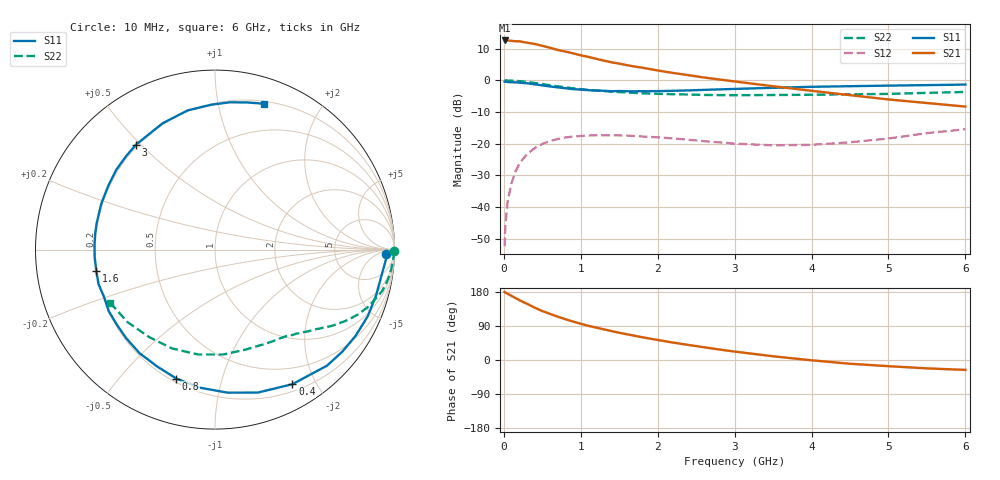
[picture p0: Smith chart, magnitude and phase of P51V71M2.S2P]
! SIEMENS Small Signal Semiconductors
! BFP183
! Si NPN RF Bipolar Junction Transistor in SOT143
! VCE = 1.75 V  IC = 1.2 mA
! Common Emitter S-Parameters:  March  1996
# GHz  S  MA  R  50
!  f  S11  S21  S12  S22
! GHz  MAG  ANG  MAG  ANG  MAG  ANG  MAG  ANG
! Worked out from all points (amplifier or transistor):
!   36 points, 10 MHz to 6 GHz, reference 50 ohm
!   highest |S21| = 12.6 dB at 10 MHz (marker M1)
!   |S21| within 3 dB of that: start of sweep to 701.4 MHz
!   unconditionally stable (mu >= 1): 2.366 GHz to end of sweep
!   at 250 MHz: K = 0.10, MSG = 18.5 dB, |S12| = -24.8 dB
!   at 1.4 GHz: K = 0.58, MSG = 11.5 dB, |S12| = -17.3 dB
!   at 6 GHz: K = 1.07, MAG = 2.0 dB, |S12| = -15.5 dB
!   S11 on the Smith chart (normalised r, x): 10 MHz: 31, -17; 400 MHz: 0.28, -1.69; 800 MHz: 0.22, -0.72; 1.6 GHz: 0.20, -0.09; 3 GHz: 0.19, +0.48; 6 GHz: 0.22, +1.37
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0.01  0.9518 -1.6  4.265 179.3  0.0024 85.2  0.9999 -0.6
0.02  0.9544 -3.2  4.259 178.4  0.0051 87.5  0.9961 -1.2
0.05  0.9405 -8.0  4.258 174.6  0.0125 85.7  0.9952 -2.8
0.1  0.9331 -15.7  4.204 169.1  0.0238 80.2  0.9891 -5.7
0.2  0.9191 -31.4  4.142 158.2  0.0475 71.5  0.9715 -11.3
0.25  0.9093 -38.7  4.037 153.0  0.0576 67.7  0.9596 -13.9
0.4  0.8651 -60.1  3.756 138.2  0.085 55.0  0.9091 -20.7
0.5  0.8315 -73.4  3.507 129.2  0.0989 47.8  0.8714 -24.7
0.6  0.8001 -85.0  3.272 121.6  0.11 41.5  0.8362 -28.0
0.7  0.7737 -96.5  3.022 114.4  0.1182 36.1  0.8044 -30.7
0.8  0.75 -106.7  2.847 107.6  0.125 31.1  0.7767 -33.2
0.9  0.7265 -116.4  2.668 101.4  0.1295 26.6  0.7494 -35.3
1.1  0.6991 -135.0  2.343 90.1  0.1343 19.0  0.7057 -39.3
1.4  0.6721 -156.7  1.929 76.3  0.1357 10.0  0.664 -44.5
1.6  0.6718 -169.6  1.737 67.9  0.1339 5.8  0.6441 -47.4
1.8  0.672 178.1  1.583 60.0  0.1297 2.6  0.6234 -50.8
2.2  0.6833 158.0  1.308 45.9  0.1209 -2.4  0.6036 -57.7
3  0.7319 127.0  0.96 22.2  0.0999 -2.4  0.582 -74.0
3.5  0.7619 112.5  0.806 9.8  0.0941 3.8  0.5863 -85.5
4.5  0.8077 91.4  0.583 -9.9  0.1051 19.0  0.6004 -113.5
5.5  0.8399 77.4  0.438 -22.1  0.1464 23.9  0.6333 -140.5
6  0.857 71.5  0.385 -26.1  0.1686 20.9  0.6549 -153.2
